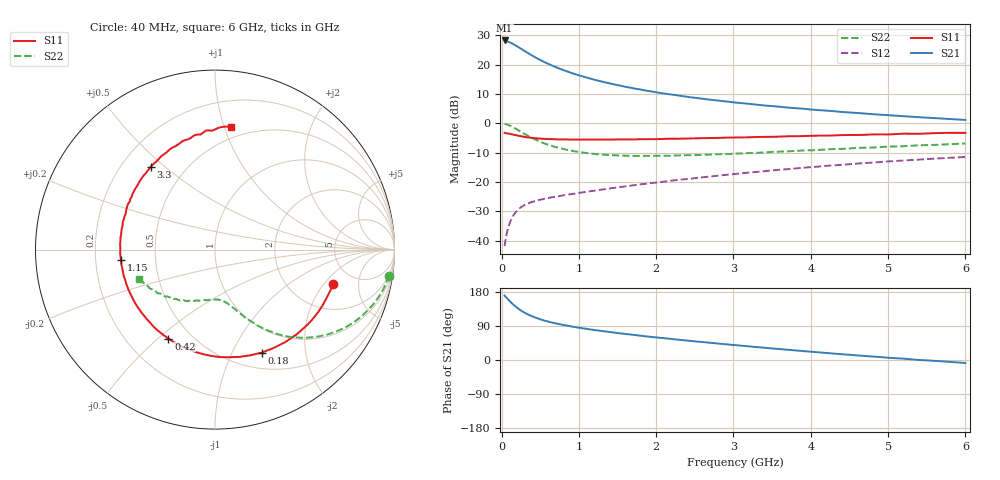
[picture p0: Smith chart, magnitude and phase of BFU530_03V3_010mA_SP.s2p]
! Filename:  P:\Prog\Test\Noise\ATS_data\Testdata_Net\03 Spar\BFU530_APG2013_40_A05_03p3V_010mA_SP_CM01_D.s2p
! Date/Time: Fri 26/Apr/2013 13:03:16
! BFU530_APG2013_40_A05_03p3V_1to25mA_SP_CM01_Bias5_R.s2p
! MDIF S-parameter v. bias file
! BFU530_APG2013_40_A05_03p3V_1to25mA_SP_CM01
! Date/time Wed Apr 24 18:17:07 2013
! VAR V_out= 3.3000
! VAR I_out= 10.0000
! VAR V_in= 0.8366
! VAR I_in= 0.1123
! Device data file deembeded for feedlines and parallel
! Original file: \03 Spar\BFU530_APG2013_40_A05_03p3V_010mA_SP_CM01_R.s2p
! Feed-files: PR047V01_250413_Feed1.s2p, PR047V01_250413_Feed2.s2p
! Parallel-file: PR047V01_250413_Par.s2p
# MHz S MA R 50
!  Freq-MHz  S11-mag  S11-arg  S21-mag  S21-arg  S12-mag  S12-arg  S22-mag  S22-arg
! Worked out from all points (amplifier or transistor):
!   98 points, 40 MHz to 6 GHz, reference 50 ohm
!   highest |S21| = 28.2 dB at 40 MHz (marker M1)
!   |S21| within 3 dB of that: start of sweep to 262.8 MHz
!   unconditionally stable (mu >= 1): 1.682 GHz to 4.046 GHz
!   at 300 MHz: K = 0.32, MSG = 26.2 dB, |S12| = -27.8 dB
!   at 1.6 GHz: K = 0.99, MSG = 17.0 dB, |S12| = -21.5 dB
!   at 6 GHz: K = 0.87, MSG = 6.3 dB, |S12| = -11.5 dB
!   S11 on the Smith chart (normalised r, x): 40 MHz: 3.49, -2.49; 180 MHz: 0.69, -1.31; 420 MHz: 0.37, -0.54; 1.15 GHz: 0.31, -0.05; 3.3 GHz: 0.32, +0.45; 6 GHz: 0.41, +1.05
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40  0.6857 -16.0  25.78 170.2  0.008073 82.8  0.9783 -8.5
50  0.6813 -20.0  25.72 167.2  0.009997 81.1  0.9723 -10.6
90  0.6683 -35.1  24.39 158.7  0.01728 74.0  0.9342 -18.9
120  0.6557 -46.1  23.54 152.4  0.02216 69.4  0.8972 -24.5
140  0.6469 -52.9  22.8 148.6  0.02506 66.6  0.8701 -28.0
180  0.6302 -65.6  21.25 141.5  0.03021 61.7  0.8139 -34.2
220  0.613 -77.2  19.82 135.1  0.03438 57.8  0.7583 -39.5
300  0.5862 -96.4  17.03 124.7  0.04066 51.9  0.6583 -47.9
360  0.5716 -108.1  15.23 118.5  0.04408 48.9  0.5961 -52.8
420  0.5595 -117.7  13.69 113.3  0.04689 47.0  0.5428 -56.5
550  0.5424 -134.5  11.13 104.3  0.05145 44.6  0.4556 -62.6
650  0.5367 -144.0  9.684 99.0  0.05481 44.0  0.4124 -66.2
800  0.5313 -155.1  8.062 92.5  0.05925 44.2  0.3646 -70.2
1050  0.5273 -169.5  6.28 83.7  0.06655 45.3  0.318 -75.5
1150  0.5273 -173.9  5.762 80.6  0.06966 45.9  0.3059 -77.2
1600  0.5308 169.1  4.195 68.7  0.08413 47.8  0.281 -85.2
2050  0.5399 156.8  3.292 58.6  0.09957 48.7  0.2791 -93.2
3100  0.5748 131.8  2.207 37.8  0.1403 47.5  0.3074 -111.7
3300  0.5845 127.7  2.078 34.1  0.1488 46.8  0.314 -115.1
4100  0.6161 112.4  1.677 20.3  0.1831 42.6  0.3512 -128.7
5200  0.666 94.1  1.321 3.5  0.2325 34.9  0.4068 -146.5
6000  0.6882 82.5  1.142 -7.9  0.2671 28.0  0.4527 -158.9
